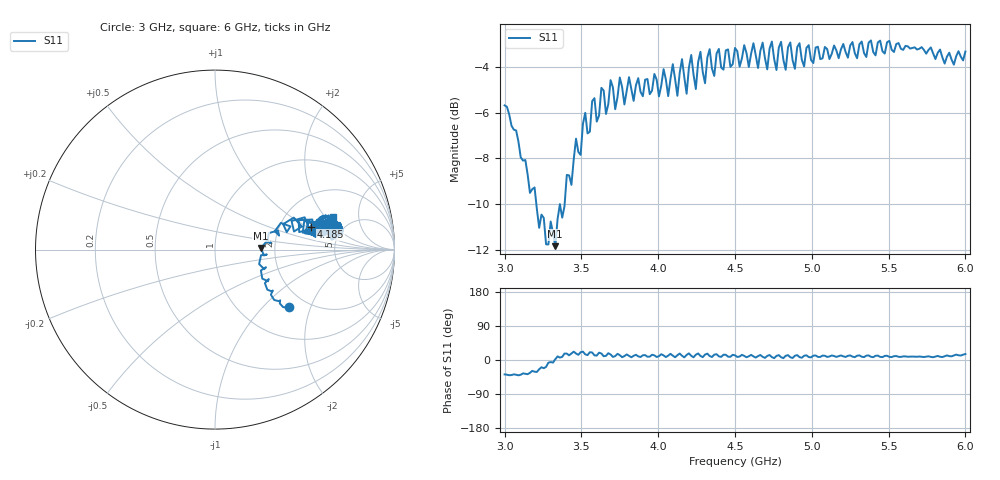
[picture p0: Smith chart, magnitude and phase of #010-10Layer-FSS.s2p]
!  05/08/2025  18:10:28
! Ref Plane: 0.000 mm
# MHZ S MA R  50
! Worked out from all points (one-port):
!   201 points, 3 GHz to 6 GHz, reference 50 ohm
!   lowest |S11| = -11.8 dB at 3.33 GHz (marker M1), VSWR 1.69, Z = 84.4 + j1.59 ohm
!   |S11| at or under -10 dB: 3.207 GHz to 3.36 GHz (152.9 MHz wide, 4.66 % of centre); 3.36 GHz to 3.391 GHz (30.53 MHz wide, 0.905 % of centre)
!   S11 on the Smith chart (normalised r, x): 3 GHz: 1.62, -1.42; 4.185 GHz: 3.01, +1.10; 6 GHz: 3.52, +2.42
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3000  0.5197 -38.0
3330  0.2563 2.0
3375  0.2957 8.3
3525  0.5006 14.9
3750  0.5979 12.7
4065  0.5444 11.5
4095  0.6393 11.5
4125  0.5454 12.7
4155  0.6556 11.2
4185  0.551 13.4
4215  0.6694 11.0
4245  0.5642 14.0
4275  0.6802 10.8
4305  0.5808 14.3
4335  0.6892 10.5
4365  0.6025 14.1
4500  0.6935 12.3
4695  0.6589 5.6
4725  0.6914 13.1
4755  0.6558 4.9
4785  0.6944 12.9
4815  0.6532 4.9
4845  0.6959 12.8
4875  0.6519 5.3
4905  0.696 12.8
5250  0.7021 12.1
5625  0.6991 8.6
6000  0.681 15.7
